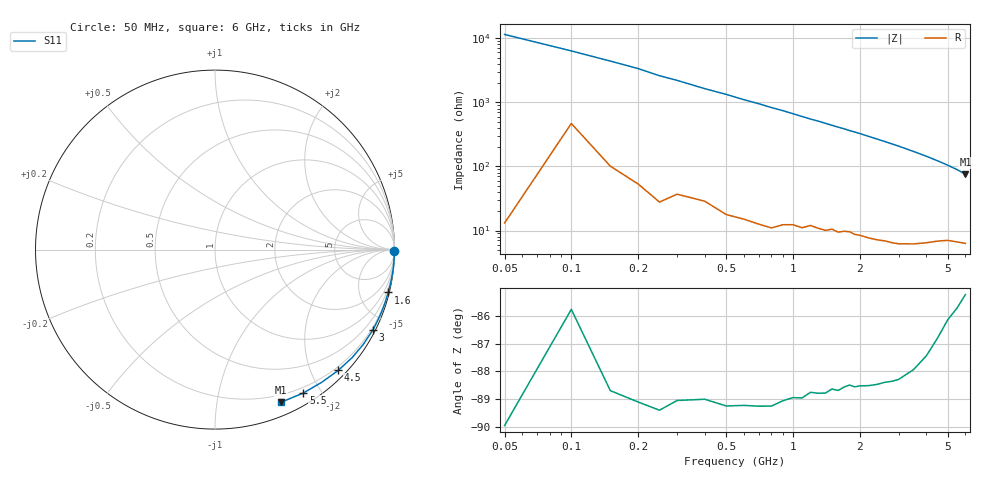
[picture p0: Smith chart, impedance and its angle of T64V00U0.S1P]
! SIEMENS Discrete & RF Semiconductors
! BAT62
! Si Schottky Diode in SOT143
! VR = 4 V
! S-Parameters:  February  1997
# GHz  S  MA  R  50
!  f  S11
! GHz  MAG  ANG
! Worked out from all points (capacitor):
!   34 points, 50 MHz to 6 GHz, reference 50 ohm
!   read as one part to ground: C = 251 fF near 50 MHz
!   lowest |Z| = 75.9 ohm at 6 GHz (marker M1)
!   S11 on the Smith chart (normalised r, x): 50 MHz: open; 1.6 GHz: 0.19, -8.20; 3 GHz: 0.12, -4.15; 4.5 GHz: 0.14, -2.44; 5.5 GHz: 0.13, -1.78; 6 GHz: 0.13, -1.51
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0.05  1 -0.5
0.1  0.9988 -0.9
0.2  0.9995 -1.7
0.25  0.9996 -2.2
0.4  0.9989 -3.5
0.5  0.999 -4.3
0.6  0.9988 -5.2
0.7  0.9986 -6.0
0.8  0.9984 -6.9
0.9  0.9978 -7.7
1.2  0.9961 -10.4
1.3  0.9959 -11.2
1.6  0.9945 -13.9
1.7  0.9936 -14.7
1.8  0.9929 -15.7
1.9  0.9928 -16.5
2  0.9923 -17.4
2.2  0.9914 -19.3
2.4  0.9903 -21.2
2.6  0.989 -23.1
2.8  0.9879 -25.1
3  0.9864 -27.1
3.5  0.9808 -32.5
4  0.9727 -38.2
4.5  0.9616 -44.4
5  0.9489 -51.1
5.5  0.9384 -58.4
6  0.9265 -66.7
